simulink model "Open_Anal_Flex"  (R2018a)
settings: Solver=ode5  StartTime=0.0  StopTime=25000  FixedStep=Ts  RelTol=1e-3  EnableMultiTasking=on
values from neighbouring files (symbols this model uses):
  Kq1 = I22*ww^2 - 3*wo2*(I11-I33)    [start.m]    (also in run.m)
  Kq2 = 2*I22*zet*ww    [start.m]    (also in run.m)
  Kqi = 0.0005    [start.m]    (also in run.m)
  Kr1 = (0.1*I11*I33*zet^2/Hy0) - sqrt( ((0.01^zet^4*I11^2*I33^2)/Hy0^2)+(4*I11*I33*zet^2) )    [start.m]    (also in run.m)
  Kr2 = 0.05*Kr1    [start.m]    (also in run.m)
  Kr3 = 0.04*zet*(Kr2-Hy0) * sqrt(abs(Hy0/(I11*I33)))    [start.m]    (also in run.m)
  Ts = 0.01    [start.m]    (also in run.m = 0.001; runf.m = 0.0005)
undefined symbols (not defined in the file or in its folder): Avf, Bvf, Cvf, den, DiscIntNeverNeededParam, dsen, Dvf, nsen, num, RW_Steering
libraries: simulink x3

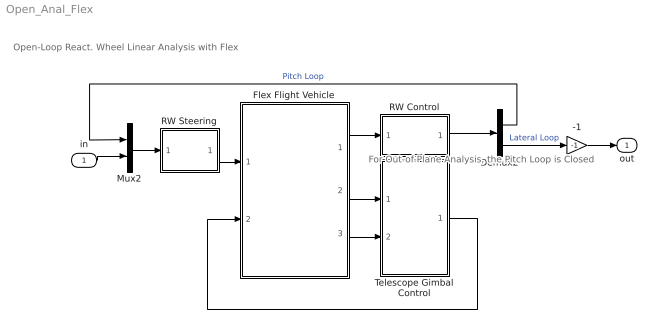
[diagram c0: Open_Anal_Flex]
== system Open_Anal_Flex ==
  note: Open-Loop React. Wheel Linear Analysis with Flex
  note: For Out-of-Plane Analysis, the Pitch Loop is Closed
  in : Inport
  -1 : Gain  Gain=-1
  Demux2 : Demux  Outputs=2
  Flex Flight Vehicle : Subsystem
  Mux2 : Mux  Inputs=2
  RW Control : Subsystem
  RW Steering : Subsystem
  Telescope Gimbal Control : Subsystem
  out : Outport
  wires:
  Flex Flight Vehicle/2(alfa) -> Telescope Gimbal Control/1(Gimb)
  Flex Flight Vehicle/3(alfad) -> Telescope Gimbal Control/2(Grate)
  Mux2/1 -> RW Steering/1(Trwc)
  Flex Flight Vehicle/1(atti) -> RW Control/1(atti)
  RW Control/1(Tc) -> Demux2/1
  RW Steering/1(Twi) -> Flex Flight Vehicle/1(Trw(i))
  Telescope Gimbal Control/1(GTrq) -> Flex Flight Vehicle/2(Tgimb)
  -1/1 -> out/1
  in/1 -> Mux2/2
  Demux2/2 -> -1/1  "Lateral Loop"
  Demux2/1 -> Mux2/1  "Pitch Loop"

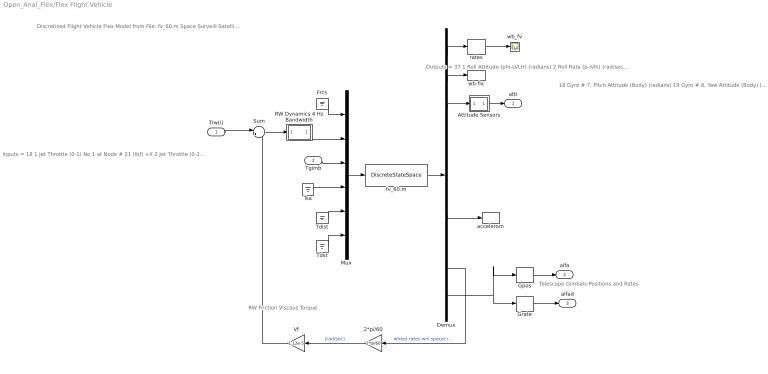
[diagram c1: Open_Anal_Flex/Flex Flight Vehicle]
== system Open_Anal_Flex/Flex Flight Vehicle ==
  note: Telescope Gimbals Positions and Rates
  note: RW Friction Viscous Torque
  note: Inputs = 18 1 Jet Throttle (0-1) No 1 at Node # 21 (lbf) +X 2 Jet Throttle (0-1) No 2 at Node # 22 (lbf) +X 3 Jet Throttle (0-1) No 3 at Node # 23 (lbf) +Y 4 Jet Throttle (0-1) No 4 at Node # 24 (lbf) -Y 5 Jet Throttle (0-1) No 5 at Node # 25 (lbf) -Y 6 Jet Throttle (0-1) No 6 at Node # 26 (lbf) +Y 7 Jet Throttle (0-1) No 7 at Node # 27 (lbf) +X 8 React-Wheel No 1 Torque to Spacecraft (ft-lb) 9 React-Wheel No 2 Torque to Spacecraft (ft-lb) 10 React-Wheel No 3 Torque to Spacecraft (ft-lb) 11 Elevation Trqu at Gimbal No 1 (ft-lb) 12 Azimuth Torque at Gimbal No 2 (ft-lb) 13 Rght SA Torque at Gimbal No 3 (ft-lb) 14 Left SA Torque at Gimbal No 4 (ft-lb) 15 Ext Torque Input 1 (ft-lb), dir: 1.00 0.00 0.00 16 Ext Torque Input 2 (ft-lb), dir: 0.00 1.00 0.00 17 Ext Torque Input 3 (ft-lb), dir: 0.00 0.00 1.00 18 Ext Torque Direct.=( 0.1970 -0.5964 -0.7782)
  note: Outputs = 37 1 Roll Attitude (phi-LVLH) (radians) 2 Roll Rate (p-lvlh) (rad/sec) 3 Pitch Attitude (thet-LVLH) (radians) 4 Pitch Rate (q-lvlh) (rad/sec) 5 Yaw Attitude (psi-LVLH) (radians) 6 Yaw Rate (r-lvlh) (rad/sec) 7 Angle of attack, alfa, (radians) 8 Angle of sideslip, beta, (radian) 9 Change in Altitude, delta-h, (feet) 10 Forward Acceleration (V-dot) (ft/sec) 11 Cross Range Velocity (Vcr) (ft/sec) 12 Rate-Gyro # 1, Roll Rate (Body) (rad/sec) 13 Rate-Gyro # 2, Pitch Rate (Body) (rad/sec) 14 Rate-Gyro # 3, Yaw Rate (Body) (rad/sec) 15 Gyro # 4, Roll Attitude (Body) (radians) 16 Gyro # 5, Pitch Attitude (Body) (radians) 17 Gyro # 6, Yaw Attitude (Body) (radians)
  note: Discretized Flight Vehicle Flex Model from File: fv_60.m Space Surveill Satellite with RCS and Reaction Wheels (Gimbals, 60 Modes, Z-Transf)
  note: 18 Gyro # 7, Pitch Attitude (Body) (radians) 19 Gyro # 8, Yaw Attitude (Body) (radians) 20 Gyro # 9, Pitch Attitude (Body) (radians) 21 Gyro # 10, Yaw Attitude (Body) (radians) 22 Gyro # 11, Roll Attitude (Body) (radians) 23 Gyro # 12, Pitch Attitude (Body) (radians) 24 Gyro # 13, Yaw Attitude (Body) (radians) 25 Translat. Accelerom # 1, (along X), (ft/sec^2) 26 Translat. Accelerom # 2, (along Y), (ft/sec^2) 27 Reaction Wheel # 1 Rate (rpm) relative to vehicle 28 Reaction Wheel # 2 Rate (rpm) relative to vehicle 29 Reaction Wheel # 3 Rate (rpm) relative to vehicle 30 Rotation Angle at Elevati Gimbal No 1 31 Rotation Rate at Elevati Gimbal No 1 32 Rotation Angle at Azimuth Gimbal No 2 33 Rotation Rate at Azimuth Gimbal No 2 34 Rotation Angle at Rght SA Gimbal No 3 35 Rotation Rate at Rght SA Gimbal No 3 36 Rotation Angle at Left SA Gimbal No 4 37 Rotation Rate at Left SA Gimbal No 4
  Trw(i) : Inport
  Tgimb : Inport  Port=2
  2*pi/60 : Gain  Gain=2*pi/60
  Attitude Sensors : Subsystem
  Demux : Demux  Outputs=[11, 3, 3, 2, 2, 3, 2, 1,2, 8]
  Frcs : Ground
  Gpos : Selector  InputPortWidth=8  IndexOptions=Index vector (dialog)  Indices=[1,3]  OutputSizes=1
  Grate : Selector  InputPortWidth=8  IndexOptions=Index vector (dialog)  Indices=[2, 4]  OutputSizes=1
  Mux : Mux  Inputs=[7,3,2,2,3,1]
  RW Dynamics 4 Hz Bandwidth : Subsystem
  Sum : Sum  Inputs=|+-
  Tdist : Ground
  Tdst : Ground
  Tsa : Ground
  Vf : Gain  Gain=1.12e-5
  accelerom : ToWorkspace  VariableName=accel  SampleTime=-1
  fv_60.m : DiscreteStateSpace  A=Avf  B=Bvf  C=Cvf  D=Dvf  SampleTime=Ts
  rates : Selector  InputPortWidth=11  IndexOptions=Index vector (dialog)  Indices=[2, 4, 6]  OutputSizes=1
  wb-flx : ToWorkspace  VariableName=wb  SampleTime=-1
  wb_fv : Scope
  atti : Outport
  alfa : Outport  Port=2
  alfad : Outport  Port=3
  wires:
  Mux/1 -> fv_60.m/1
  Demux/9 -> 2*pi/60/1  "wheel rates wrt spacecrft (rpm)"
  Demux/1 -> rates/1
  rates/1 -> wb_fv/1
  Demux/10 -> Gpos/1, Grate/1
  Demux/2 -> wb-flx/1
  Demux/7 -> accelerom/1
  Demux/3 -> Attitude Sensors/1(I)
  Grate/1 -> alfad/1
  Gpos/1 -> alfa/1
  Tsa/1 -> Mux/4
  Tdst/1 -> Mux/6
  Tdist/1 -> Mux/5
  Vf/1 -> Sum/2
  2*pi/60/1 -> Vf/1  "(rad/sec)"
  Tgimb/1 -> Mux/3
  fv_60.m/1 -> Demux/1
  Trw(i)/1 -> Sum/1
  Sum/1 -> RW Dynamics 4 Hz Bandwidth/1(I)
  RW Dynamics 4 Hz Bandwidth/1(O) -> Mux/2
  Attitude Sensors/1(O) -> atti/1
  Frcs/1 -> Mux/1

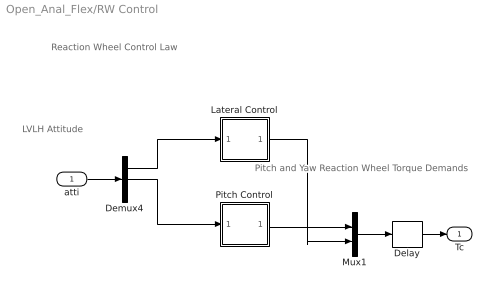
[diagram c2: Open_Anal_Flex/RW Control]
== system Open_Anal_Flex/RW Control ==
  note: Pitch and Yaw Reaction Wheel Torque Demands
  note: LVLH Attitude
  note: Reaction Wheel Control Law
  atti : Inport
  Delay : Delay  DelayLength=1  InputProcessing=Inherited  SampleTime=Ts
  Demux4 : Demux  Outputs=3
  Lateral Control : Subsystem
  Mux1 : Mux  Inputs=2
  Pitch Control : Subsystem
  Tc : Outport
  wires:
  Demux4/1 -> Lateral Control/1(phi)
  Pitch Control/1(Tcy) -> Mux1/1
  Demux4/2 -> Pitch Control/1(the)
  atti/1 -> Demux4/1
  Mux1/1 -> Delay/1
  Lateral Control/1(Tcz) -> Mux1/2
  Delay/1 -> Tc/1

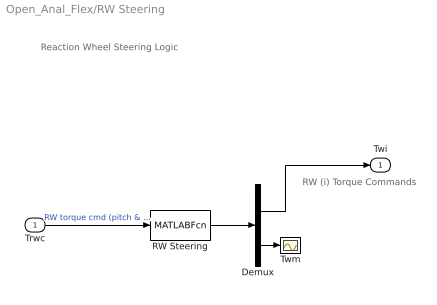
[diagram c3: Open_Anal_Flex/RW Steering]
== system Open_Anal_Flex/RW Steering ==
  note: Reaction Wheel Steering Logic
  note: RW (i) Torque Commands
  Trwc : Inport
  Demux : Demux  Outputs=[2, 1]
  RW Steering : MATLABFcn  MATLABFcn=RW_Steering( u(1:2) )  OutputDimensions=3
  Twm : Scope
  Twi : Outport
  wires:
  Trwc/1 -> RW Steering/1  "RW torque cmd (pitch & yaw)"
  RW Steering/1 -> Demux/1
  Demux/1 -> Twi/1
  Demux/2 -> Twm/1

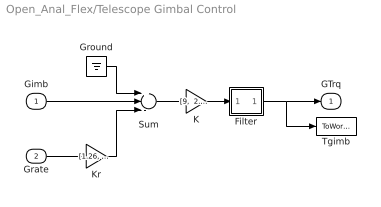
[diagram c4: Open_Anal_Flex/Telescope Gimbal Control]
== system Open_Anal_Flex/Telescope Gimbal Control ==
  Gimb : Inport
  Grate : Inport  Port=2
  Filter : Subsystem
  Ground : Ground
  K : Gain  Gain="[9,  2.85]"
  Kr : Gain  Gain="[1.26,  1.14]"
  Sum : Sum  Inputs=+--
  Tgimb : ToWorkspace  VariableName=Tgimb  SampleTime=-1
  GTrq : Outport
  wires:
  Filter/1(O) -> Tgimb/1, GTrq/1
  Ground/1 -> Sum/1
  Kr/1 -> Sum/3
  K/1 -> Filter/1(I)
  Grate/1 -> Kr/1
  Gimb/1 -> Sum/2
  Sum/1 -> K/1

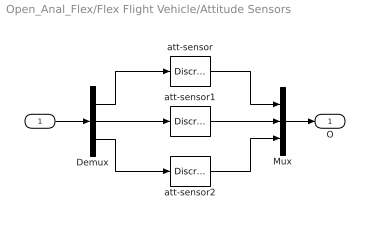
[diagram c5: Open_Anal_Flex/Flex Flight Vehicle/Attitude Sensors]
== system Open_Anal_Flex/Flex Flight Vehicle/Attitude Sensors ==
  I : Inport
  Demux : Demux  Outputs=3
  Mux : Mux  Inputs=3
  att-sensor : DiscreteTransferFcn  Numerator=[nsen]  Denominator=[dsen]  SampleTime=Ts
  att-sensor1 : DiscreteTransferFcn  Numerator=[nsen]  Denominator=[dsen]  SampleTime=Ts
  att-sensor2 : DiscreteTransferFcn  Numerator=[nsen]  Denominator=[dsen]  SampleTime=Ts
  O : Outport
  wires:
  I/1 -> Demux/1
  Mux/1 -> O/1
  att-sensor/1 -> Mux/1
  Demux/1 -> att-sensor/1
  Demux/3 -> att-sensor2/1
  att-sensor2/1 -> Mux/3
  Demux/2 -> att-sensor1/1
  att-sensor1/1 -> Mux/2

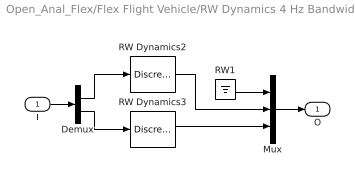
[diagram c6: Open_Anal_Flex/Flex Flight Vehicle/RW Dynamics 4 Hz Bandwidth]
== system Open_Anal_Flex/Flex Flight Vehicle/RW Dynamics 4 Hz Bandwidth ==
  I : Inport
  Demux : Demux  Outputs=2
  Mux : Mux  Inputs=3
  RW Dynamics2 : DiscreteTransferFcn  Numerator="[0  0.221199217]"  Denominator=[1 -0.778800783]  SampleTime=Ts
  RW Dynamics3 : DiscreteTransferFcn  Numerator="[0  0.221199217]"  Denominator=[1 -0.778800783]  SampleTime=Ts
  RW1 : Ground
  O : Outport
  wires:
  Demux/2 -> RW Dynamics3/1
  Demux/1 -> RW Dynamics2/1
  RW Dynamics2/1 -> Mux/2
  RW Dynamics3/1 -> Mux/3
  I/1 -> Demux/1
  Mux/1 -> O/1
  RW1/1 -> Mux/1

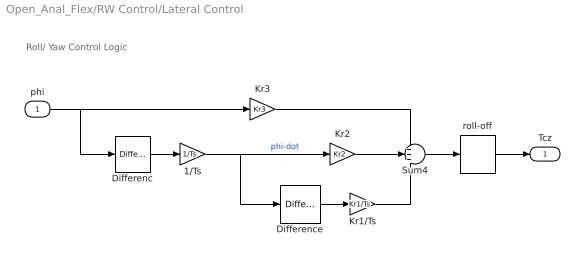
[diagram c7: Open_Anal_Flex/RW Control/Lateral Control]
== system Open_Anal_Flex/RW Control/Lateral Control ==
  note: Roll/ Yaw Control Logic
  phi : Inport
  1/Ts : Gain  Gain=1/Ts
  Differenc : simulink/Discrete/Difference  ICPrevInput=0.0  InputProcessing=Inherited  OutMin=[]  OutMax=[]  OutDataType=sfix(16)  OutScaling=2^-10  DoSatur=off
  Difference : simulink/Discrete/Difference  ICPrevInput=0.0  InputProcessing=Inherited  OutMin=[]  OutMax=[]  OutDataType=sfix(16)  OutScaling=2^-10  DoSatur=off
  Kr1/Ts : Gain  Gain=Kr1/Ts
  Kr2 : Gain  Gain=Kr2
  Kr3 : Gain  Gain=Kr3
  Sum4 : Sum  Inputs=+++
  roll-off : DiscreteTransferFcn  Numerator=[num]  Denominator=[den]  SampleTime=Ts
  Tcz : Outport
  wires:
  roll-off/1 -> Tcz/1
  Kr3/1 -> Sum4/1
  Kr2/1 -> Sum4/2
  Kr1/Ts/1 -> Sum4/3
  phi/1 -> Kr3/1, Differenc/1
  Sum4/1 -> roll-off/1
  Difference/1 -> Kr1/Ts/1
  Differenc/1 -> 1/Ts/1
  1/Ts/1 -> Kr2/1, Difference/1  "phi-dot"

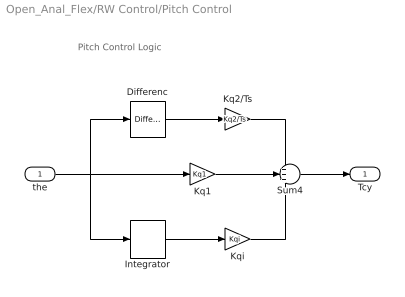
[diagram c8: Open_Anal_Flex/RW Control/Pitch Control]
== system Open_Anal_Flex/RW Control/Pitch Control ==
  note: Pitch Control Logic
  the : Inport
  Differenc : simulink/Discrete/Difference  ICPrevInput=0.0  InputProcessing=Inherited  OutMin=[]  OutMax=[]  OutDataType=sfix(16)  OutScaling=2^-10  DoSatur=off
  Integrator : DiscreteIntegrator  SampleTime=Ts  ICPrevOutput=DiscIntNeverNeededParam  ICPrevScaledInput=DiscIntNeverNeededParam
  Kq1 : Gain  Gain=Kq1
  Kq2/Ts : Gain  Gain=Kq2/Ts
  Kqi : Gain  Gain=Kqi
  Sum4 : Sum  Inputs=+++
  Tcy : Outport
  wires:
  Kq1/1 -> Sum4/2
  Sum4/1 -> Tcy/1
  Kq2/Ts/1 -> Sum4/1
  the/1 -> Kq1/1, Integrator/1, Differenc/1
  Kqi/1 -> Sum4/3
  Integrator/1 -> Kqi/1
  Differenc/1 -> Kq2/Ts/1

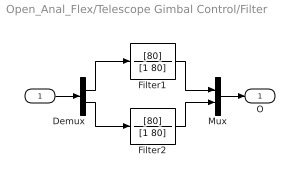
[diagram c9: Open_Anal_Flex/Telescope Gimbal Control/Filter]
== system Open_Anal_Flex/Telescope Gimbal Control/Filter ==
  I : Inport
  Demux : Demux  Outputs=2
  Filter1 : TransferFcn  Numerator=[80]  Denominator=[1 80]
  Filter2 : TransferFcn  Numerator=[80]  Denominator=[1 80]
  Mux : Mux  Inputs=2
  O : Outport
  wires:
  Filter1/1 -> Mux/1
  Filter2/1 -> Mux/2
  Demux/1 -> Filter1/1
  Demux/2 -> Filter2/1
  I/1 -> Demux/1
  Mux/1 -> O/1
